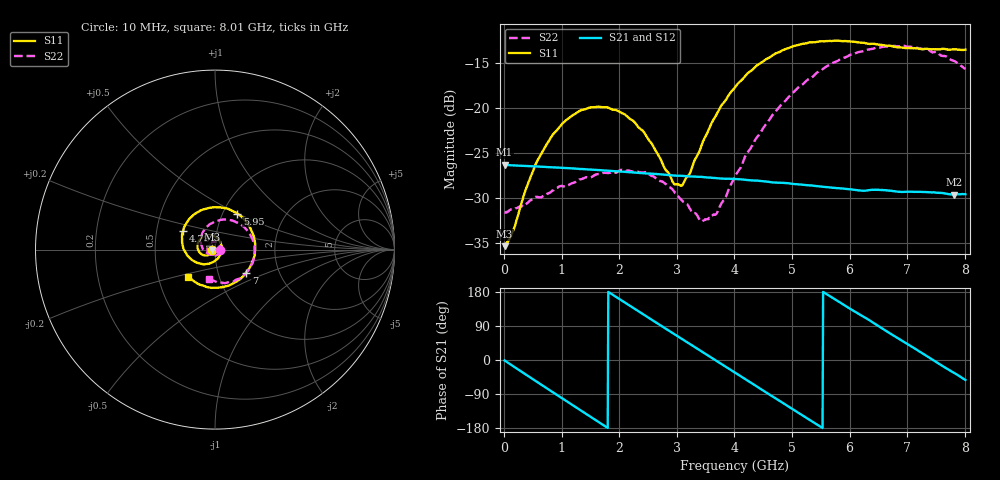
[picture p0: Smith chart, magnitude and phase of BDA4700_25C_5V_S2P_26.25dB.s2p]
!Agilent Technologies,E5071B,MY42404982,A.09.10
!Date: Mon Oct 20 13:39:42 2025
!Data & Calibration Information:
!Freq	S11:SOLT2(ON)	S21:SOLT2(ON)	S12:SOLT2(ON)	S22:SOLT2(ON)
# Hz S RI R 50
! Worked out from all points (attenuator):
!   801 points, 10 MHz to 8.01 GHz, reference 50 ohm
!   highest |S21| = -26.32 dB at 10 MHz (marker M1); lowest = -29.7 dB at 7.82 GHz (marker M2)
!   lowest |S11| = -35.4 dB at 10 MHz (marker M3), VSWR 1.03, Z = 48.3 - j0.105 ohm
!   |S11| at or under -10 dB: start of sweep to end of sweep
!   |S22| runs from -32.7 to -13.0 dB; largest |S21 - S12| = 0.0004
!   S11 on the Smith chart (normalised r, x): 10 MHz: 0.97, -0.00; 4.78 GHz: 0.68, +0.15; 5.95 GHz: 1.17, +0.50; 7 GHz: 1.37, -0.37; 8.01 GHz: 0.71, -0.22
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1e7  -0.0169 -0.00109  0.0483 -0.00103  0.0483 -0.00107  0.0261 -0.000787
1.5e8  -0.0181 -0.00957  0.0462 -0.0128  0.0462 -0.0128  0.0264 -0.00718
4.1e8  -0.0277 -0.0253  0.0356 -0.0315  0.0356 -0.0315  0.0203 -0.0215
7e8  -0.0496 -0.0331  0.0157 -0.0443  0.0157 -0.0443  0.00593 -0.0321
1.03e9  -0.08 -0.0221  -0.0106 -0.0452  -0.0106 -0.0452  -0.0164 -0.0327
1.35e9  -0.0974 0.00811  -0.0323 -0.0324  -0.0323 -0.0324  -0.0361 -0.0178
2.08e9  -0.0486 0.0792  -0.0395 0.0199  -0.0394 0.0199  -0.0297 0.0336
2.68e9  0.0262 0.0479  -0.00366 0.0426  -0.00369 0.0426  0.0129 0.0374
2.94e9  0.037 0.00984  0.0145 0.0396  0.0146 0.0395  0.0251 0.024
3.09e9  0.0341 -0.0144  0.0238 0.0345  0.0237 0.0345  0.0279 0.0124
3.41e9  0.00319 -0.0594  0.0376 0.0173  0.0376 0.0172  0.0204 -0.0117
3.54e9  -0.0169 -0.0722  0.0401 0.0086  0.0401 0.00849  0.0129 -0.0203
3.7e9  -0.0481 -0.0802  0.0406 -0.00234  0.0406 -0.00245  -0.000757 -0.0261
4.01e9  -0.112 -0.0675  0.0337 -0.022  0.0337 -0.0219  -0.0323 -0.0259
4.78e9  -0.1785 0.1025  -0.0116 -0.0366  -0.0114 -0.0366  -0.0787 0.0641
5.35e9  -0.066 0.2235  -0.0352 -0.0112  -0.0352 -0.0113  -0.0155 0.148
5.95e9  0.1252 0.2004  -0.0274 0.0224  -0.0275 0.0223  0.1192 0.1523
6.68e9  0.2217 -0.0238  0.0106 0.033  0.0106 0.033  0.2202 0.000254
7e9  0.1745 -0.128  0.0251 0.0231  0.0252 0.0231  0.2029 -0.0859
7.43e9  0.0433 -0.2083  0.0338 0.00102  0.034 0.000932  0.1193 -0.1678
7.82e9  -0.0949 -0.1903  0.0271 -0.0187  0.0271 -0.0188  0.0152 -0.1823
8.01e9  -0.1494 -0.1501  0.0201 -0.0263  0.0201 -0.0263  -0.0309 -0.1622
